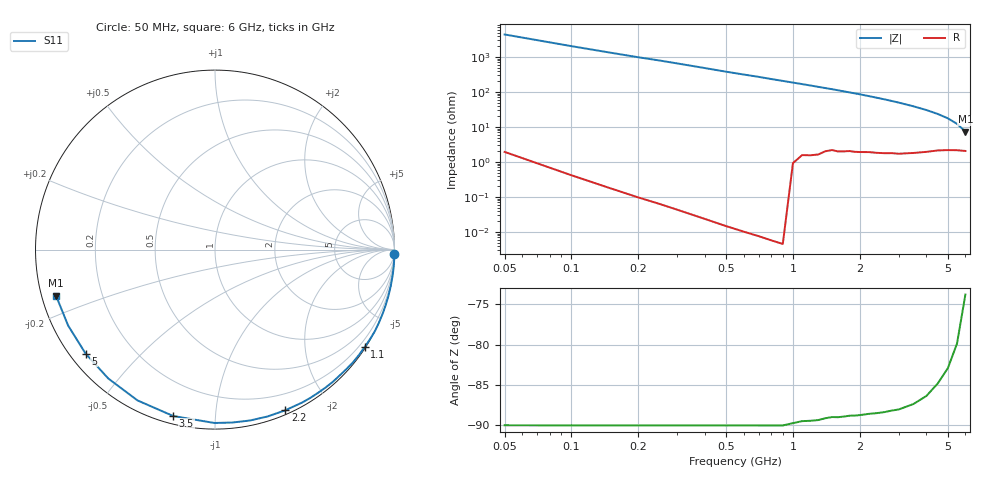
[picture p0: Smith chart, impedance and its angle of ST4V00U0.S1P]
! SIEMENS Discrete & RF Semiconductors
! BA892
! Si PIN Diode in SCD-80
! VR = 4 V
! S-Parameters:  September  1997
# GHz  S  MA  R  50
!  f  S11
! GHz  MAG  ANG
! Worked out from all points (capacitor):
!   34 points, 50 MHz to 6 GHz, reference 50 ohm
!   read as one part to ground: C = 778 fF near 50 MHz
!   lowest |Z| = 7.4 ohm at 6 GHz (marker M1)
!   S11 on the Smith chart (normalised r, x): 50 MHz: 0, -88; 1.1 GHz: 0.03, -3.36; 2.2 GHz: 0.04, -1.53; 3.5 GHz: 0.04, -0.78; 5 GHz: 0.04, -0.35; 6 GHz: 0.04, -0.14
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0.05  1 -1.3
0.25  1 -7.2
0.4  1 -11.8
0.5  1 -15.0
0.6  1 -18.0
0.7  1 -20.9
0.8  1 -24.1
0.9  1 -27.1
1.1  0.9949 -33.1
1.2  0.994 -36.1
1.3  0.9927 -39.2
1.4  0.9896 -42.2
1.5  0.9872 -45.1
1.6  0.9868 -48.2
1.7  0.985 -51.3
1.9  0.9822 -57.3
2  0.9808 -60.3
2.2  0.9772 -66.4
2.4  0.9748 -72.5
2.6  0.9719 -78.4
2.8  0.9683 -84.3
3  0.966 -90.2
3.5  0.9559 -104.1
4  0.9448 -117.2
4.5  0.9324 -129.6
5  0.925 -141.2
5.5  0.9213 -152.7
6  0.9221 -163.8
